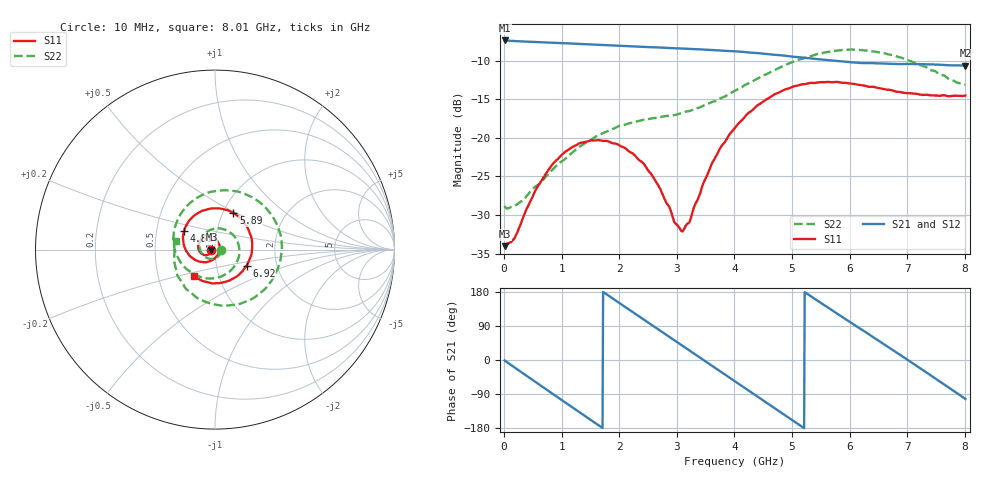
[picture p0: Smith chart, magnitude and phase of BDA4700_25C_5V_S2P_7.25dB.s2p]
!Agilent Technologies,E5071B,MY42404982,A.09.10
!Date: Mon Oct 20 13:29:36 2025
!Data & Calibration Information:
!Freq	S11:SOLT2(ON)	S21:SOLT2(ON)	S12:SOLT2(ON)	S22:SOLT2(ON)
# Hz S RI R 50
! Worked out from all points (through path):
!   801 points, 10 MHz to 8.01 GHz, reference 50 ohm
!   highest |S21| = -7.36 dB at 20 MHz (marker M1); lowest = -10.6 dB at 8.01 GHz (marker M2)
!   group delay of S21, straight-line fit = 285 ps
!   lowest |S11| = -34.0 dB at 10 MHz (marker M3), VSWR 1.04, Z = 48.1 - j0.0849 ohm
!   |S11| at or under -10 dB: start of sweep to end of sweep
!   |S22| runs from -29.2 to -8.5 dB; largest |S21 - S12| = 0.0034
!   S11 on the Smith chart (normalised r, x): 10 MHz: 0.96, -0.00; 4.81 GHz: 0.69, +0.15; 5.89 GHz: 1.12, +0.48; 6.92 GHz: 1.40, -0.26; 8.01 GHz: 0.76, -0.23
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1e7  -0.0198 -0.000883  0.4282 -0.00918  0.4284 -0.0096  0.0361 -0.00286
2e7  -0.0202 -0.00165  0.428 -0.0168  0.4278 -0.0181  0.0354 -0.00326
3.4e8  -0.025 -0.0184  0.3397 -0.2498  0.3398 -0.2503  0.023 -0.0327
7.2e8  -0.0491 -0.031  0.0987 -0.404  0.0988 -0.4042  -0.0198 -0.052
1.02e9  -0.0756 -0.0222  -0.1242 -0.3921  -0.1244 -0.3924  -0.0625 -0.0341
1.35e9  -0.0931 0.00647  -0.3198 -0.2502  -0.3199 -0.2502  -0.0865 0.0228
1.64e9  -0.0887 0.0387  -0.3977 -0.0553  -0.3977 -0.0553  -0.0654 0.0807
1.93e9  -0.066 0.064  -0.3675 0.1495  -0.3675 0.1496  -0.00518 0.1158
2.32e9  -0.0218 0.0699  -0.1812 0.3459  -0.1811 0.346  0.0909 0.0905
2.68e9  0.014 0.0469  0.0629 0.3806  0.0627 0.3805  0.1358 -9.26e-05
3.11e9  0.0238 -0.00754  0.3058 0.2245  0.305 0.2253  0.0868 -0.1172
3.55e9  -0.0152 -0.0582  0.3679 -0.0577  0.368 -0.0584  -0.0479 -0.16
4.01e9  -0.0978 -0.0629  0.2012 -0.3034  0.2013 -0.3033  -0.1866 -0.0783
4.4e9  -0.1624 -0.00494  -0.0418 -0.3523  -0.0419 -0.3526  -0.2316 0.071
4.81e9  -0.1723 0.1015  -0.2593 -0.2246  -0.2584 -0.2256  -0.1597 0.24
5.35e9  -0.068 0.2169  -0.3172 0.0795  -0.3173 0.0788  0.0961 0.3269
5.89e9  0.103 0.203  -0.1154 0.291  -0.1156 0.2906  0.3356 0.1581
6.27e9  0.1856 0.1137  0.0822 0.2942  0.085 0.2929  0.3642 -0.06
6.68e9  0.2042 -0.0189  0.2533 0.1652  0.254 0.165  0.2397 -0.2523
6.92e9  0.1758 -0.0889  0.2974 0.0482  0.2972 0.0471  0.1183 -0.3071
7.59e9  0.000204 -0.188  0.1521 -0.2563  0.1514 -0.2569  -0.1968 -0.1637
8.01e9  -0.1174 -0.1469  -0.0649 -0.2867  -0.0646 -0.2871  -0.2163 0.048
